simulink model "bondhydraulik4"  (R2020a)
settings: Solver=ode45  StartTime=0.0  StopTime=2  RelTol=1e-3  EnableMultiTasking=on
undefined symbols (not defined in the file or in its folder): Display, Int, libbondgraph
libraries: libbondgraph x9

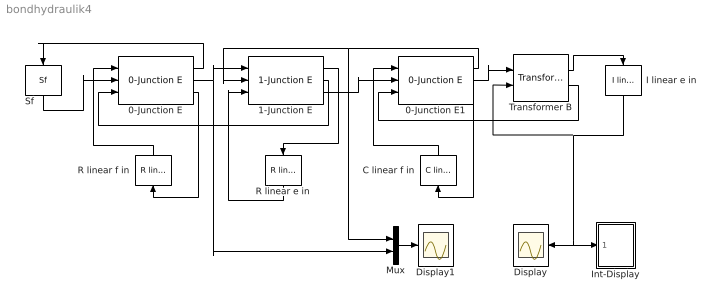
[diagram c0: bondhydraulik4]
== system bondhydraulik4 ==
  0-Junction E : libbondgraph/0-Junction E
  0-Junction E1 : libbondgraph/0-Junction E
  1-Junction E : libbondgraph/1-Junction E
  C linear f in : libbondgraph/C linear f in  C=1.74e-12
  Display : Scope
  Display1 : Scope
  I linear e in : libbondgraph/I linear e in  I=500
  Int-Display : Subsystem  AncestorBlock=libbondgraph/Int-Display
  Mux : Mux  Inputs=2
  R linear e in : libbondgraph/R linear e in  R=8e7
  R linear f in : libbondgraph/R linear f in  R=1e9
  Sf : libbondgraph/Sf  f_ext=0.001
  Transformer B : libbondgraph/Transformer B  m=1000
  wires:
  Sf/1 -> 0-Junction E/2
  0-Junction E/1 -> Sf/1
  0-Junction E/3 -> R linear f in/1
  R linear f in/1 -> 0-Junction E/1
  0-Junction E/2 -> 1-Junction E/1, Mux/2
  1-Junction E/2 -> 0-Junction E/3
  Transformer B/1 -> I linear e in/1
  I linear e in/1 -> Transformer B/2, Display/1, Int-Display/1(In1)
  Mux/1 -> Display1/1
  1-Junction E/1 -> R linear e in/1
  R linear e in/1 -> 1-Junction E/3
  1-Junction E/3 -> 0-Junction E1/2
  0-Junction E1/1 -> 1-Junction E/2, Mux/1
  0-Junction E1/3 -> C linear f in/1
  C linear f in/1 -> 0-Junction E1/1
  0-Junction E1/2 -> Transformer B/1
  Transformer B/2 -> 0-Junction E1/3

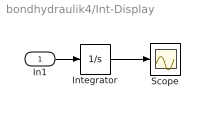
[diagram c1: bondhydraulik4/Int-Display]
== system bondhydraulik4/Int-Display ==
  In1 : Inport
  Integrator : Integrator
  Scope : Scope
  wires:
  In1/1 -> Integrator/1
  Integrator/1 -> Scope/1
